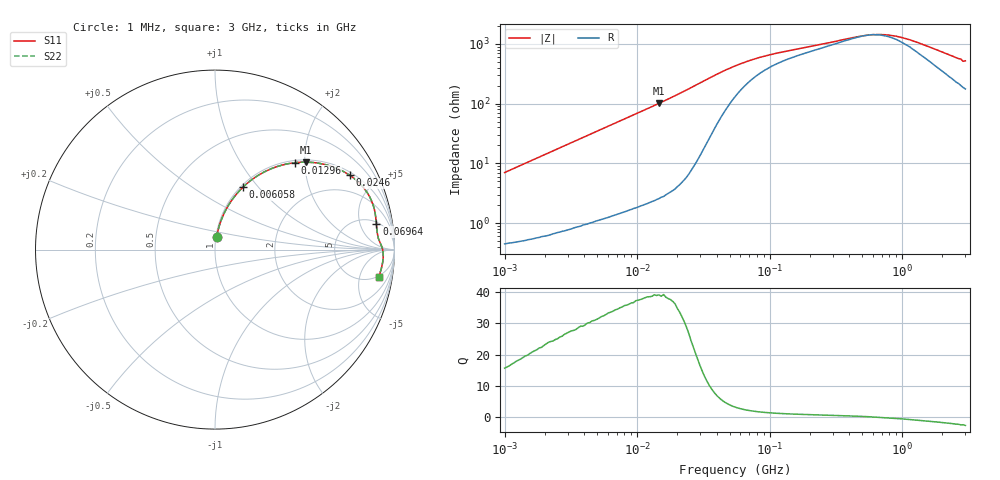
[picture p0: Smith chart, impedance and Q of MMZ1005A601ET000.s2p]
! S-parameter Generated by TDK Corporation
! Copyright(C) 2016 TDK Corporation.
! All Rights Reserved.
! TDK P/N: MMZ1005A601ET000 (Chip Beads)
! Property: |Z|=600¶ at 100MHz
! Size(LxWxT): 1x0.5x0.5mm, 0.039x0.02x0.02inches
! Model Type: s2p (Touchstone File Format Version 1.0)
! Frequency: DC=Yes Start=1MHz Stop=3000MHz 202points Log-sweep
! Note: This model was converted from impedance.
! Model Generated on May. 16, 2016
! Hash(MD5):
! Port Assignments:
!  1 ---@@@--- 2
! Applicable Conditions:
!  Temperature = 25 degC
!  DC Bias Current = 0 A
!  Small Signal Operation
! Terms and conditions regarding TDK Simulation Models
! (1)This simulation model is being provided solely for informational purposes. Please refer to the specifications of the products in terms of detailed characteristics of such products.
! (2)In no event shall TDK Corporation of any of its subsidiaries be liable for any loss or damage arising, directly or indirectly,
!  From any information contained in this simulation model, including, but not limited to loss or damages arising from any inaccuracies, omissions or errors in connection with such information.
! (3)Any and all copyrights on this simulation model are owned by TDK Corporation.
!  Duplication or redistribution of this simulation model without prior written permission from TDK Corporation is prohibited.
! (4)This simulation model is subject to any modification or change without any prior notice.
! (5)Neither TDK Corporation nor any of its subsidiaries shall make any warranty, express or implied,
!  Including but not limited to the correctness, implied warranties of merchantability and fitness for a particular purpose with respect to this simulation models.
! (6)The use of this simulation model shall be deemed to have consented to the terms and conditions hereof.
# MHz S MA R 50
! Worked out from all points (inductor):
!   201 points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, 1 MHz to 3 GHz, reference 50 ohm
!   read as one part in series: L = 1.12 uH near 1.041 MHz
!   highest Q = 39.2 at 14.62 MHz (marker M1), where L = 1.1 uH
!   self-resonance near 571.1 MHz
!   S11 on the Smith chart (normalised r, x): 1 MHz: 1.01, +0.14; 6.058 MHz: 1.03, +0.84; 12.96 MHz: 1.05, +1.79; 24.6 MHz: 1.13, +3.55; 69.64 MHz: 6, +9; 3 GHz: 5, -10
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1  0.07 82.3  0.9931 -4.0  0.9931 -4.0  0.07 82.3
2.055611  0.1416 79.4  0.9839 -8.1  0.9839 -8.1  0.1416 79.4
3.900413  0.2592 73.0  0.957 -15.0  0.957 -15.0  0.2592 73.0
6.058321  0.3817 65.9  0.9129 -22.4  0.9129 -22.4  0.3817 65.9
8.686058  0.5071 58.0  0.848 -30.5  0.848 -30.5  0.5071 58.0
12.9622  0.6585 47.4  0.7358 -41.2  0.7358 -41.2  0.6585 47.4
14.61624  0.7025 43.9  0.694 -44.6  0.694 -44.6  0.7025 43.9
18.58443  0.7833 36.9  0.6009 -51.5  0.6009 -51.5  0.7833 36.9
24.59509  0.858 28.8  0.4825 -59.0  0.4825 -59.0  0.858 28.8
28.86629  0.8874 24.4  0.4144 -62.4  0.4144 -62.4  0.8874 24.4
35.26298  0.9086 19.5  0.336 -64.7  0.336 -64.7  0.9086 19.5
54.77226  0.9139 11.7  0.2136 -60.5  0.2136 -60.5  0.9139 11.7
69.64249  0.9107 9.0  0.1744 -54.8  0.1744 -54.8  0.9107 9.0
108.1723  0.9088 5.8  0.1327 -43.8  0.1327 -43.8  0.9088 5.8
213.6344  0.9159 3.1  0.09889 -30.2  0.09889 -30.2  0.9159 3.1
515.4121  0.9327 0.4  0.06756 -5.3  0.06756 -5.3  0.9327 0.4
655.3423  0.9356 -0.5  0.06505 7.8  0.06505 7.8  0.9356 -0.5
800.5644  0.9372 -1.4  0.06685 19.4  0.06685 19.4  0.9372 -1.4
1147.801  0.9381 -3.0  0.0801 37.9  0.0801 37.9  0.9381 -3.0
2769.173  0.9279 -8.9  0.1663 59.9  0.1663 59.9  0.9279 -8.9
2882.277  0.9203 -9.6  0.1798 59.0  0.1798 59.0  0.9203 -9.6
3000  0.9258 -9.6  0.1777 60.6  0.1777 60.6  0.9258 -9.6
